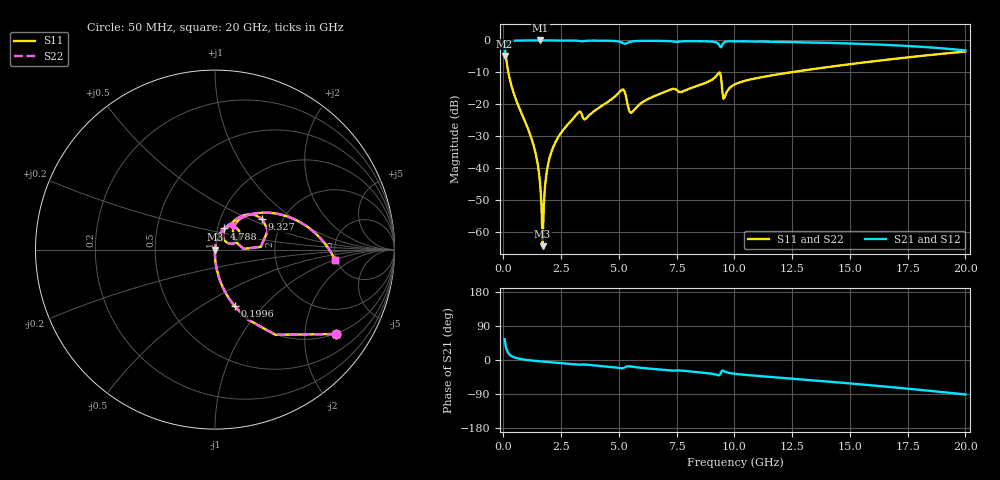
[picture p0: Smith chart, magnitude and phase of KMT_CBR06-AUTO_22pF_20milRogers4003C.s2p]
! Data measured by Modelithics Inc. support@modelithics.com 813-866-6335
! KEMET CBR06-AUTO 22pF, Pad Width= 0.851mm, Pad Length= 0.64mm, Pad Gap= 0.62mm, 20mil Rogers 4003C substrate Data, January 2022
# hz S ma R 50
! 2 Port Network Data from SP1.SP block
! freq  magS11  angS11  magS21  angS21  magS12  angS12  magS22  angS22
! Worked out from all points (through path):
!   401 points, 50 MHz to 20 GHz, reference 50 ohm
!   highest |S21| = -0.01 dB at 1.596 GHz (marker M1); lowest = -4.9 dB at 50 MHz (marker M2)
!   group delay of S21, straight-line fit = 13 ps
!   lowest |S11| = -64.4 dB at 1.696 GHz (marker M3), VSWR 1.00, Z = 50.1 - j0.00198 ohm
!   |S11| at or under -10 dB: 212.9 MHz to 12.42 GHz (12.21 GHz wide, 193 % of centre)
!   |S22| runs from -64.4 to -1.7 dB; largest |S21 - S12| = 0
!   S11 on the Smith chart (normalised r, x): 50 MHz: 0.99, -2.86; 199.6 MHz: 0.99, -0.71; 4.788 GHz: 1.08, +0.26; 9.327 GHz: 1.58, +0.60; 20 GHz: 4.85, -0.97
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5e7  0.8203 -35.0  0.5716 55.0  0.5716 55.0  0.8203 -35.0
1.99625e8  0.3343 -70.9  0.9421 19.0  0.9421 19.0  0.3343 -70.9
5.4875e8  0.1166 -84.5  0.9928 5.3  0.9928 5.3  0.1166 -84.5
1.34675e9  0.01995 -90.7  0.9992 -2.2  0.9992 -2.2  0.01995 -90.7
1.496375e9  0.01081 -90.1  0.9993 -3.1  0.9993 -3.1  0.01081 -90.1
1.596125e9  0.005251 -87.3  0.9993 -3.6  0.9993 -3.6  0.005251 -87.3
1.695875e9  0.0006027 -1.9  0.9993 -4.2  0.9993 -4.2  0.0006027 -1.9
1.795625e9  0.005038 78.2  0.9993 -4.7  0.9993 -4.7  0.005038 78.2
1.94525e9  0.01209 81.4  0.9992 -5.5  0.9992 -5.5  0.01209 81.4
2.194625e9  0.02313 81.4  0.9989 -6.7  0.9989 -6.7  0.02313 81.4
3.192125e9  0.07106 71.6  0.9894 -11.9  0.9894 -11.9  0.07106 71.6
3.391625e9  0.06954 53.9  0.9695 -12.0  0.9695 -12.0  0.06954 53.9
4.788125e9  0.129 66.1  0.9809 -19.2  0.9809 -19.2  0.129 66.1
5.187125e9  0.1703 38.3  0.9026 -21.2  0.9026 -21.2  0.1703 38.3
5.53625e9  0.07402 43.6  0.9618 -17.3  0.9618 -17.3  0.07402 43.6
6.73325e9  0.144 62.8  0.9833 -24.8  0.9833 -24.8  0.144 62.8
9.32675e9  0.3135 32.9  0.8631 -40.4  0.8631 -40.4  0.3135 32.9
9.576125e9  0.1284 38.5  0.9462 -30.4  0.9462 -30.4  0.1284 38.5
1.0025e10  0.2061 51.4  0.9707 -36.5  0.9707 -36.5  0.2061 51.4
1.336662e10  0.3547 35.5  0.9279 -53.5  0.9279 -53.5  0.3547 35.5
1.670825e10  0.5043 17.1  0.8471 -71.1  0.8471 -71.1  0.5043 17.1
2e10  0.6698 -4.7  0.6974 -90.8  0.6974 -90.8  0.6698 -4.7
